(* Logix 5000 DataType export VMAC_DATA_MSG; software revision 30.00 *)

TYPE VMAC_DATA_MSG :
STRUCT
   STATUS : CONNECTION_STATUS;
   DATA : DINT[100];
   LEN : DINT;
   ROUNDS : DINT;
   VMAC : DINT[8];
END_STRUCT
END_TYPE
